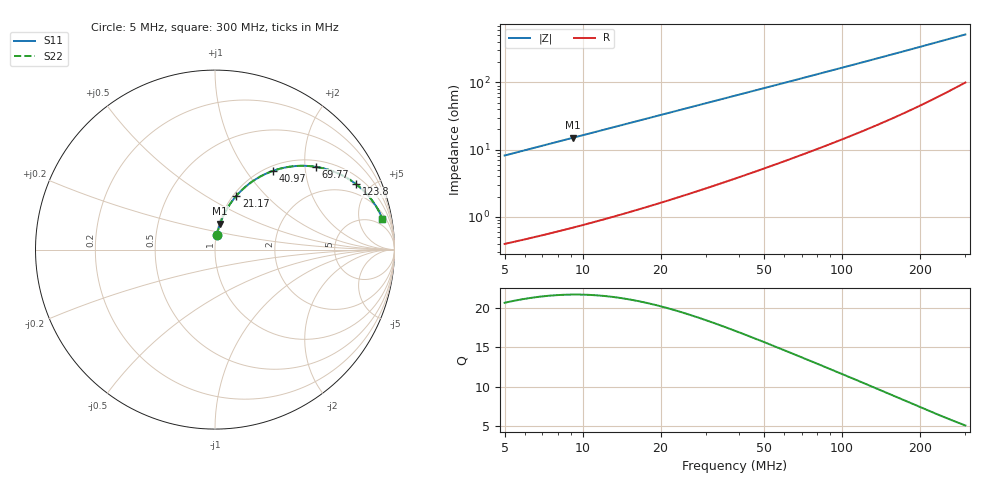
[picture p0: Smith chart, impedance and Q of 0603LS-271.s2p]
# MHz S MA R 50
!Freq  MagS11  AngS11  MagS21  AngS21  MagS12  AngS12  MagS22  AngS22
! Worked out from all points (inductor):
!   801 points, 5 MHz to 300 MHz, reference 50 ohm
!   read as one part in series: L = 261 nH near 5.103 MHz
!   highest Q = 21.6 at 9.193 MHz (marker M1), where L = 261 nH
!   S11 on the Smith chart (normalised r, x): 5 MHz: 1.01, +0.16; 21.17 MHz: 1.03, +0.69; 40.97 MHz: 1.08, +1.34; 69.77 MHz: 1.17, +2.29; 123.8 MHz: 1.40, +4.09; 300 MHz: 3, +10
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5  0.08139 82.6  0.9927 -4.7  0.9927 -4.7  0.08139 82.6
6.937805  0.1124 80.9  0.9884 -6.4  0.9884 -6.4  0.1124 80.9
9.19327  0.148 78.9  0.9822 -8.5  0.9822 -8.5  0.148 78.9
11.63359  0.1857 76.6  0.974 -10.7  0.974 -10.7  0.1857 76.6
14.42337  0.2277 74.1  0.963 -13.1  0.963 -13.1  0.2277 74.1
17.60968  0.2738 71.4  0.9486 -15.9  0.9486 -15.9  0.2738 71.4
21.17231  0.3229 68.3  0.9304 -18.8  0.9304 -18.8  0.3229 68.3
25.32576  0.3765 64.9  0.907 -22.1  0.907 -22.1  0.3765 64.9
29.98549  0.432 61.3  0.8787 -25.6  0.8787 -25.6  0.432 61.3
35.14103  0.4874 57.6  0.8459 -29.1  0.8459 -29.1  0.4874 57.6
40.97276  0.543 53.8  0.808 -32.8  0.808 -32.8  0.543 53.8
47.28577  0.5953 50.0  0.7672 -36.4  0.7672 -36.4  0.5953 50.0
54.29291  0.6447 46.2  0.7232 -40.0  0.7232 -40.0  0.6447 46.2
69.76777  0.7281 39.3  0.6346 -46.6  0.6346 -46.6  0.7281 39.3
85.61748  0.7869 33.8  0.5577 -51.7  0.5577 -51.7  0.7869 33.8
103.467  0.8321 29.0  0.4867 -56.0  0.4867 -56.0  0.8321 29.0
123.7645  0.8668 24.9  0.4222 -59.6  0.4222 -59.6  0.8668 24.9
152.6604  0.898 20.5  0.3525 -63.2  0.3525 -63.2  0.898 20.5
175.2826  0.9137 18.0  0.3108 -65.1  0.3108 -65.1  0.9137 18.0
202.2899  0.9266 15.6  0.2714 -66.7  0.2714 -66.7  0.9266 15.6
252.0866  0.9408 12.5  0.2186 -68.2  0.2186 -68.2  0.9408 12.5
300  0.9483 10.4  0.1834 -68.5  0.1834 -68.5  0.9483 10.4
